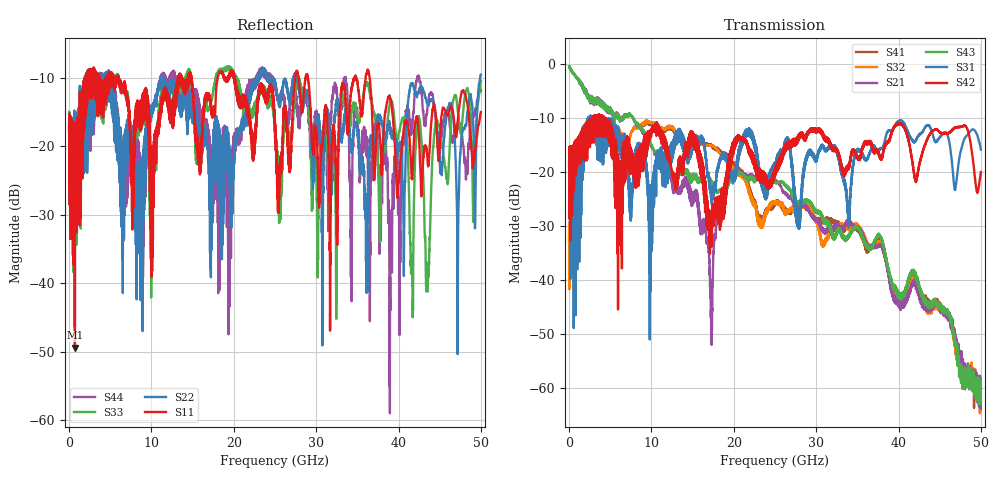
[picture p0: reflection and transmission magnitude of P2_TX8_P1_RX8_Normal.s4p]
!Keysight Technologies,N5225A,MY51441389,A.10.49.11
!Date: Monday, July 08, 2019 15:06:10
!Correction: S11(Full 4 Port(1,2,3,4))
!S12(Full 4 Port(1,2,3,4))
!S13(Full 4 Port(1,2,3,4))
!S14(Full 4 Port(1,2,3,4))
!S21(Full 4 Port(1,2,3,4))
!S22(Full 4 Port(1,2,3,4))
!S23(Full 4 Port(1,2,3,4))
!S24(Full 4 Port(1,2,3,4))
!S31(Full 4 Port(1,2,3,4))
!S32(Full 4 Port(1,2,3,4))
!S33(Full 4 Port(1,2,3,4))
!S34(Full 4 Port(1,2,3,4))
!S41(Full 4 Port(1,2,3,4))
!S42(Full 4 Port(1,2,3,4))
!S43(Full 4 Port(1,2,3,4))
!S44(Full 4 Port(1,2,3,4))
!S4P File: Measurements: <S11,S12,S13,S14>,
!<S21,S22,S23,S24>,
!<S31,S32,S33,S34>,
!<S41,S42,S43,S44>:
# Hz S  dB  R 50
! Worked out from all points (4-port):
!   5000 points, 10 MHz to 50 GHz, reference 50 ohm
!   strongest paths, dB at 10 MHz, 12.51 GHz, 25.01 GHz, 37.51 GHz, 50 GHz:
!     S42: -19.1, -20.4, -20.7, -16.3, -20.0
!     S31: -19.1, -16.2, -18.3, -15.9, -15.9
!     S43: -0.4, -20.3, -22.0, -31.8, -59.8
!     S21: -0.4, -22.0, -21.6, -33.8, -63.9
!     S32: -32.9, -11.6, -25.9, -33.2, -62.0
!     S41: -32.7, -11.9, -26.1, -32.7, -60.1
!   lowest |S11| = -49.4 dB at 710 MHz (marker M1), VSWR 1.01, Z = 49.8 - j0.287 ohm
!   |S11| at or under -10 dB: 6.036 GHz to 13.22 GHz (7.183 GHz wide, 74.6 % of centre); 20.08 GHz to 27.44 GHz (7.364 GHz wide, 31 % of centre); 36.49 GHz to end of sweep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
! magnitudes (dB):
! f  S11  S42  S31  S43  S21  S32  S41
! 10 MHz  -17.7  -19.1  -19.1  -0.4  -0.4  -32.9  -32.7
! 710 MHz  -49.4  -20.7  -26.4  -2.0  -2.0  -18.9  -18.9
! 17.26 GHz  -14.8  -32.8  -23.8  -21.6  -51.2  -15.1  -14.9
! 20.34 GHz  -12.5  -14.7  -18.5  -19.8  -19.3  -20.1  -18.9
! 36.14 GHz  -9.4  -14.9  -17.9  -33.5  -33.1  -33.0  -34.4
! 43.51 GHz  -21.9  -13.8  -11.3  -44.9  -45.6  -46.0  -44.1
! 50 GHz  -15.0  -20.0  -15.9  -59.8  -63.9  -62.0  -60.1
